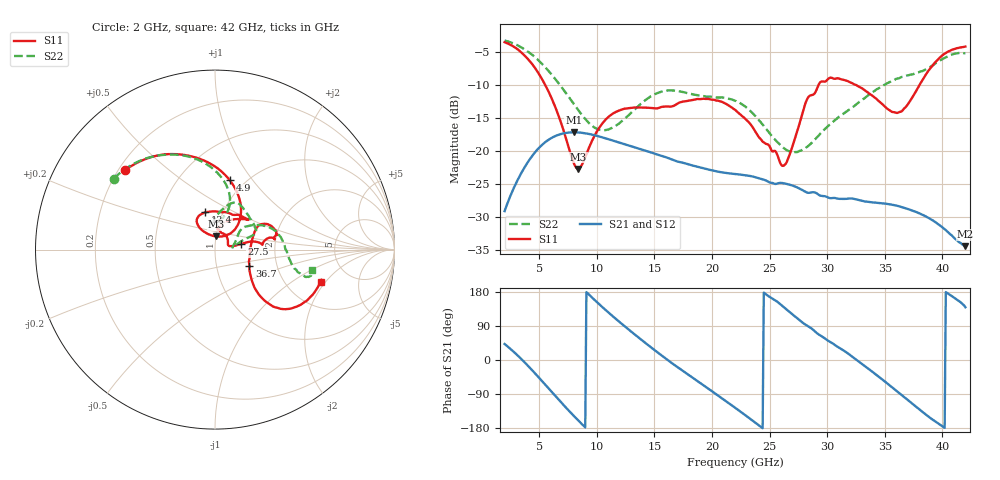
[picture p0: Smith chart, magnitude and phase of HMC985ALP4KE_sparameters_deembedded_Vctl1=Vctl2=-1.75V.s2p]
!s2p File: Measurements: S11, S21, S12, S22
# GHz S dB R 50.0
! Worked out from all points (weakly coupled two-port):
!   401 points, 2 GHz to 42 GHz, reference 50 ohm
!   highest |S21| = -17.14 dB at 8 GHz (marker M1); lowest = -34.4 dB at 42 GHz (marker M2)
!   lowest |S11| = -22.7 dB at 8.4 GHz (marker M3), VSWR 1.16, Z = 50.1 + j7.37 ohm
!   |S11| at or under -10 dB: 5.531 GHz to 29.25 GHz (23.72 GHz wide, 136 % of centre); 32.53 GHz to 38.01 GHz (5.481 GHz wide, 15.5 % of centre)
!   |S22| runs from -20.2 to -3.2 dB; largest |S21 - S12| = 0.00015
!   S11 on the Smith chart (normalised r, x): 2 GHz: 0.23, +0.36; 4.9 GHz: 0.85, +0.78; 13.4 GHz: 0.83, +0.36; 27.5 GHz: 1.34, +0.09; 36.7 GHz: 1.44, -0.27; 42 GHz: 3.11, -1.81
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2  -3.50 138.4  -29.07 42.2  -29.07 42.2  -3.24 144.9
3.4  -4.97 110.0  -23.47 4.1  -23.47 4.1  -4.23 121.6
4.9  -8.08 77.9  -19.65 -43.9  -19.66 -43.9  -6.18 97.6
6.2  -12.47 53.1  -17.87 -88.1  -17.88 -88.1  -8.64 80.7
8  -21.78 63.8  -17.14 -147.3  -17.14 -147.3  -12.83 71.7
8.4  -22.68 84.9  -17.17 -159.7  -17.17 -159.8  -13.80 73.0
8.7  -22.10 100.2  -17.21 -168.9  -17.22 -168.9  -14.49 74.7
10.8  -15.16 124.5  -18.07 131.0  -18.07 131.0  -16.80 93.2
13.4  -13.39 104.3  -19.47 64.8  -19.48 64.8  -13.49 82.8
15.4  -13.45 78.3  -20.59 17.3  -20.59 17.3  -11.10 69.3
18.9  -12.12 42.8  -22.44 -58.9  -22.45 -58.9  -11.59 43.6
22  -13.74 55.6  -23.45 -125.8  -23.46 -125.8  -12.36 21.8
24.5  -18.67 83.0  -24.32 177.7  -24.32 177.7  -16.16 17.6
26.2  -22.22 18.7  -24.85 140.3  -24.85 140.3  -19.48 8.8
27.5  -16.42 12.3  -25.57 107.3  -25.57 107.3  -20.05 8.2
28.7  -11.49 5.9  -26.22 81.9  -26.22 81.8  -18.64 19.0
31.1  -9.06 18.1  -27.22 31.3  -27.22 31.3  -14.70 37.8
33.3  -10.82 28.9  -27.62 -16.8  -27.61 -16.8  -11.91 32.3
35.4  -13.78 8.8  -28.03 -66.2  -28.02 -66.2  -9.57 21.1
36.7  -13.51 -24.8  -28.59 -98.2  -28.59 -98.2  -8.69 12.2
39.6  -6.15 -42.1  -30.98 -166.7  -30.99 -166.6  -6.52 -14.6
42  -4.16 -16.8  -34.38 139.3  -34.35 139.2  -5.16 -11.8
